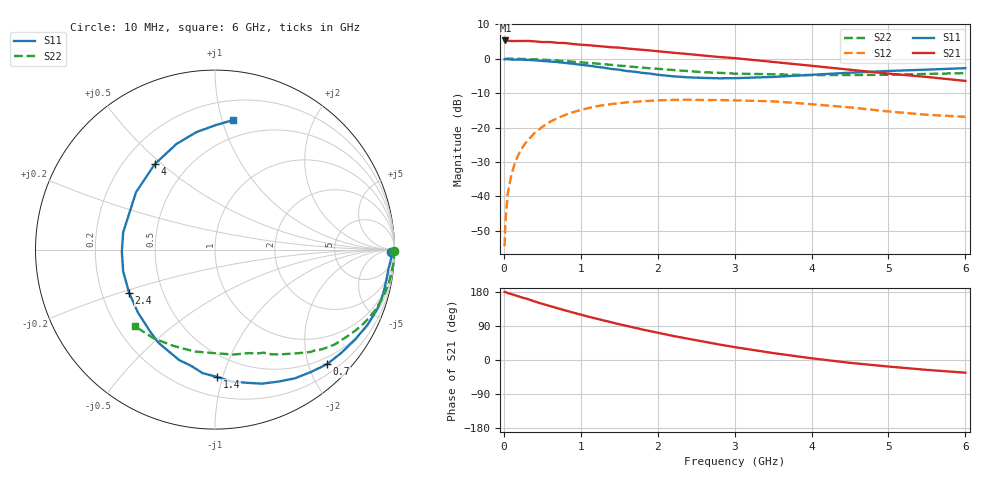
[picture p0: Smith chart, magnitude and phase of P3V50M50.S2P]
! SIEMENS Small Signal Semiconductors
! BFP181
! Si NPN RF Bipolar Junction Transistor in SOT143
! VCE = 0.5 V  IC = 0.5 mA
! Common Emitter S-Parameters:  March  1996
# GHz  S  MA  R  50
!  f  S11  S21  S12  S22
! GHz  MAG  ANG  MAG  ANG  MAG  ANG  MAG  ANG
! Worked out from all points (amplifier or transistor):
!   36 points, 10 MHz to 6 GHz, reference 50 ohm
!   highest |S21| = 5.3 dB at 20 MHz (marker M1)
!   |S21| within 3 dB of that: start of sweep to 1.942 GHz
!   unconditionally stable (mu >= 1): 3.327 GHz to end of sweep
!   at 250 MHz: K = 0.10, MSG = 15.3 dB, |S12| = -25.5 dB
!   at 1.4 GHz: K = 0.51, MSG = 8.2 dB, |S12| = -13.1 dB
!   at 6 GHz: K = 1.72, MAG = 0.3 dB, |S12| = -16.9 dB
!   S11 on the Smith chart (normalised r, x): 10 MHz: 61, -44; 700 MHz: 0.37, -2.33; 1.4 GHz: 0.34, -0.96; 2.4 GHz: 0.32, -0.21; 4 GHz: 0.33, +0.47; 6 GHz: 0.35, +1.09
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0.01  0.9787 -0.9  1.834 179.7  0.0019 89.3  0.9997 -0.3
0.02  0.9834 -1.4  1.839 179.5  0.0042 91.9  0.9951 -0.6
0.05  0.982 -3.0  1.823 176.8  0.0109 90.4  0.9982 -1.8
0.1  0.9723 -6.7  1.803 173.8  0.0211 84.9  0.9983 -3.5
0.15  0.9699 -9.9  1.805 170.6  0.0321 82.5  0.9948 -5.3
0.2  0.9687 -13.4  1.809 167.3  0.0425 80.7  0.9931 -7.1
0.3  0.963 -19.9  1.814 161.6  0.0634 75.9  0.9866 -10.6
0.4  0.9475 -26.3  1.783 154.5  0.0835 70.9  0.978 -14.0
0.7  0.8931 -45.6  1.699 136.5  0.1377 57.2  0.9381 -23.9
0.8  0.8667 -51.9  1.687 130.7  0.153 52.9  0.9228 -26.9
1.1  0.7923 -70.5  1.57 114.3  0.1922 40.6  0.8671 -35.5
1.4  0.7101 -88.9  1.463 99.5  0.2201 29.5  0.8134 -43.1
1.5  0.6918 -95.7  1.448 94.4  0.2252 26.5  0.7923 -45.0
1.8  0.6222 -114.6  1.345 80.5  0.2411 18.0  0.7427 -50.9
2.2  0.5545 -140.7  1.22 63.5  0.252 6.9  0.6853 -58.4
2.4  0.5357 -153.3  1.166 55.9  0.2538 1.8  0.6603 -62.0
3  0.5206 169.4  1.019 34.0  0.248 -11.0  0.6072 -71.7
3.5  0.5438 144.0  0.897 18.3  0.2404 -19.1  0.5939 -79.9
4  0.5825 125.2  0.789 4.5  0.2184 -26.5  0.5772 -90.2
4.5  0.6267 110.0  0.691 -7.5  0.1964 -32.6  0.579 -101.6
5.5  0.6934 89.7  0.543 -26.1  0.1535 -34.2  0.601 -124.4
6  0.729 82.0  0.476 -33.5  0.1432 -31.1  0.6173 -136.1
